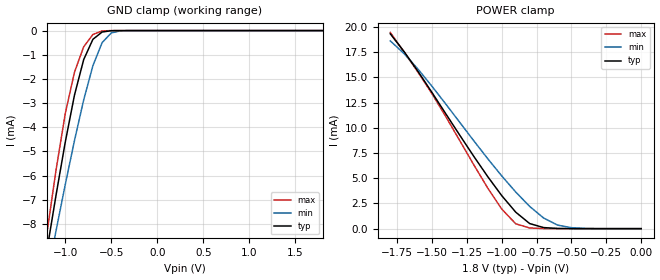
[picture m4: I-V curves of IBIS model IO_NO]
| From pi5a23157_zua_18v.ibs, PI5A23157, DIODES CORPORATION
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[Model]   IO_NO
Model_type   Terminator
C_comp   3.078pF   3.046pF   3.195pF
[Voltage Range]   1.8   1.65   1.95
[Temperature Range]   25   -40   125
[GND Clamp Reference]   0   0   0
[POWER Clamp Reference]   1.8   1.65   1.95
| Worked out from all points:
|   GND clamp passes 1 mA (typ) near -0.78 V on its own axis
|   POWER clamp passes 1 mA (typ) near -0.84 V on its own axis
[GND_Clamp]
-1.8V     -43.97mA   -353.4mA   -25.26mA
-1.2V     -9.098mA   -10.25mA   -8.383mA
-1.1V     -6.79mA    -8.263mA   -5.753mA
-1V       -4.605mA   -6.359mA   -3.421mA
-900mV    -2.662mA   -4.541mA   -1.717mA
-800mV    -1.198mA   -2.865mA   -669.7uA
-700mV    -360.7uA   -1.451mA   -161.7uA
-600mV    -59.18uA   -497.6uA   -14.42uA
-500mV    -5.324uA   -97.48uA   -563nA
-400mV    -315.9nA   -10.75uA   -13.07nA
1.8V      267.9pA    72.57nA    181.9pA
[Power_Clamp]
-1.8V     19.33mA    18.63mA    19.47mA
-1.7V     17.55mA    17.35mA    17.5mA
-1.5V     13.49mA    14.11mA    13.37mA
-1.1V     5.146mA    6.927mA    4.014mA
-1V       3.269mA    5.225mA    1.939mA
-900mV    1.637mA    3.634mA    481.1uA
-800mV    504.8uA    2.208mA    68.25uA
-700mV    107.2uA    1.056mA    7.789uA
-600mV    18.47uA    353.6uA    572.5nA
-500mV    1.916uA    98.22uA    23.25nA
-400mV    132.7nA    19.45uA    1.284nA
0V        268.2pA    3.121nA    282.8pA
